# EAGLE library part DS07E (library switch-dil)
DIL/CODE SWITCH
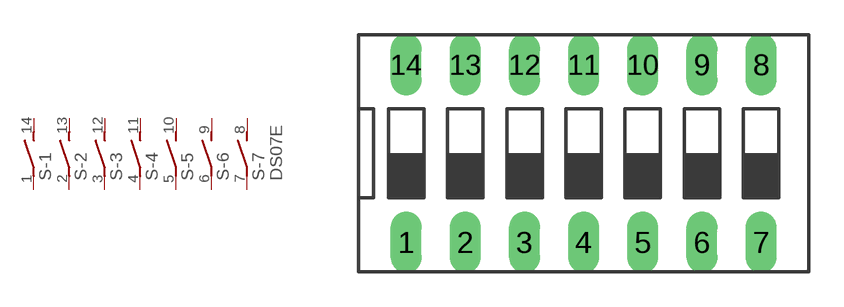
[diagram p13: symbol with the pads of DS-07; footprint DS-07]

Designator prefix S; gates -1=S -2=S -3=S -4=S -5=S -6=S -7=S+V

## DS07E (MPN: MCDS07; OC_FARNELL: 1255226; OC_NEWARK: 26M1106)  [DS-07]
1  -1:1  pas
2  -2:1  pas
3  -3:1  pas
4  -4:1  pas
5  -5:1  pas
6  -6:1  pas
7  -7:1  pas
8  -7:2  pas
9  -6:2  pas
10  -5:2  pas
11  -4:2  pas
12  -3:2  pas
13  -2:2  pas
14  -1:2  pas

## Footprint DS-07 (pad centres in mm)
DIL/CODE SWITCH Mors distributor Buerklin, 17G560
drill 0.813 long: 1 -7.62,-3.81; 2 -5.08,-3.81; 3 -2.54,-3.81; 4 0,-3.81; 5 2.54,-3.81; 6 5.08,-3.81; 7 7.62,-3.81; 8 7.62,3.81; 9 5.08,3.81; 10 2.54,3.81; 11 0,3.81; 12 -2.54,3.81; 13 -5.08,3.81; 14 -7.62,3.81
